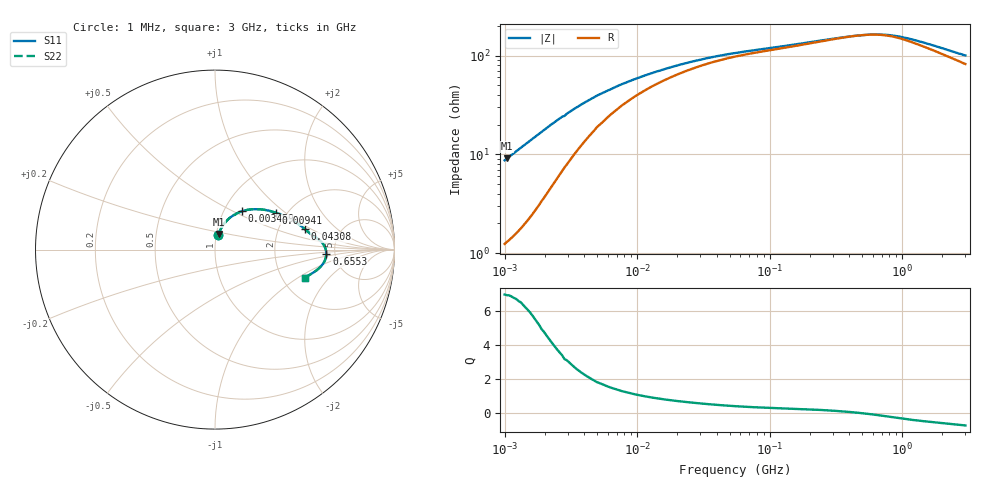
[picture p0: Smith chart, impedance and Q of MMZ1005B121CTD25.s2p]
! S-Parameter Data Generated by TDK Corporation
! Copyright(C) 2025 TDK Corporation.
! All Rights Reserved.
! TDK P/N: MMZ1005B121CTD25 (Chip Bead)
! Property: |Z|=120ohm at 100MHz
! Size(LxWxT): 1x0.5x0.5mm
! Model Type: s2p (Touchstone File Format Version 1.0)
! Frequency: DC=Yes Start=1MHz Stop=3000MHz 202points Log-sweep
! Model Generated on Feb. 6, 2025
! Terms and conditions regarding TDK Simulation Models:
! 1)This simulation model is being provided solely for informational
!  purposes. Please refer to the specifications of the products in
!  terms of detailed characteristics of such products.
! 2)In no event shall TDK Corporation of any of its subsidiaries be
!  liable for any loss or damage arising, directly or indirectly,
!  from any information contained in this simulation model, including,
!  but not limited to loss or damages arising from any inaccuracies,
!  omissions or errors in connection with such information.
! 3)Any and all copyrights on this simulation model are owned by
!  TDK Corporation.  Duplication or redistribution of this simulation
!  model without prior written permission from TDK Corporation
!  is prohibited.
! 4)This simulation model is subject to any modification or change
!  without any prior notice.
! 5)Neither TDK Corporation nor any of its subsidiaries shall make any
!  warranty, express or implied, including but not limited to the
!  correctness, implied warranties of merchantability and fitness for
!  a particular purpose with respect to this simulation models.
! 6)The use of this simulation model shall be deemed to have consented
!  to the terms and conditions hereof.
! Port Assignments:
!  1 ---@@@--- 2
! Applicable Conditions:
!  Temperature = 25 degC
!  DC Bias Current = 0 A
!  Small Signal Operation
# Hz S MA R 50
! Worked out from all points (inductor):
!   201 points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, 1 MHz to 3 GHz, reference 50 ohm
!   read as one part in series: L = 1.38 uH near 1.041 MHz
!   highest Q = 6.9 at 1.041 MHz (marker M1), where L = 1.37 uH
!   self-resonance near 518.2 MHz
!   S11 on the Smith chart (normalised r, x): 1 MHz: 1.02, +0.17; 3.459 MHz: 1.21, +0.55; 9.41 MHz: 1.76, +0.86; 43.08 MHz: 2.81, +0.87; 655.3 MHz: 4.25, -0.32; 3 GHz: 2.64, -1.15
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1000000  0.0857 76.9  0.9842 -4.9  0.9842 -4.9  0.0857 76.9
1040844  0.0893 76.7  0.9833 -5.1  0.9833 -5.1  0.0893 76.7
1492300  0.1281 73.4  0.9711 -7.3  0.9711 -7.3  0.1281 73.4
1974946  0.1675 68.7  0.9521 -9.4  0.9521 -9.4  0.1675 68.7
2720446  0.2201 61.4  0.9152 -12.2  0.9152 -12.2  0.2201 61.4
2831560  0.2229 60.2  0.9101 -12.3  0.9101 -12.3  0.2229 60.2
2947212  0.233 59.3  0.9037 -12.8  0.9037 -12.8  0.233 59.3
3459026  0.26 55.1  0.8774 -14.1  0.8774 -14.1  0.26 55.1
3900413  0.2797 51.8  0.8558 -14.9  0.8558 -14.9  0.2797 51.8
4959344  0.3172 45.2  0.8085 -16.2  0.8085 -16.2  0.3172 45.2
6058321  0.344 40.5  0.7717 -16.8  0.7717 -16.8  0.344 40.5
9410094  0.3958 31.3  0.6931 -17.3  0.6931 -17.3  0.3958 31.3
1.461624e7  0.4384 24.2  0.6264 -16.7  0.6264 -16.7  0.4384 24.2
2.559965e7  0.4825 17.5  0.5588 -15.0  0.5588 -15.0  0.4825 17.5
4.307715e7  0.5135 12.8  0.5122 -12.9  0.5122 -12.9  0.5135 12.8
5.477226e7  0.525 11.2  0.4956 -11.9  0.4956 -11.9  0.525 11.2
2.136344e8  0.5832 5.3  0.4228 -7.4  0.4228 -7.4  0.5832 5.3
3.894533e8  0.6085 2.1  0.3925 -3.3  0.3925 -3.3  0.6085 2.1
6.553423e8  0.6208 -2.1  0.3804 3.5  0.3804 3.5  0.6208 -2.1
8.005644e8  0.6192 -4.2  0.3851 6.7  0.3851 6.7  0.6192 -4.2
1.347129e9  0.5932 -9.6  0.4267 13.4  0.4267 13.4  0.5932 -9.6
3e9  0.525 -17.5  0.5237 17.5  0.5237 17.5  0.525 -17.5
